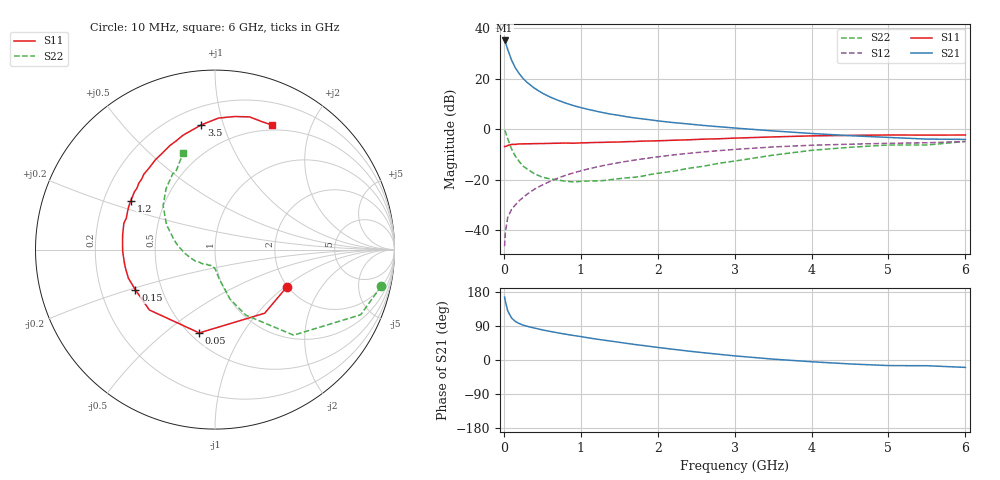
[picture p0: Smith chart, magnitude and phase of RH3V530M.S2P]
! SIEMENS Small Signal Semiconductors
! BFR106
! Si NPN RF Bipolar Junction Transistor in SOT23
! VCE = 3.5 V  IC = 30 mA
! Common Emitter S-Parameters:  August  1996
# GHz  S  MA  R  50
!  f  S11  S21  S12  S22
! GHz  MAG  ANG  MAG  ANG  MAG  ANG  MAG  ANG
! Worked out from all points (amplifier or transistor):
!   36 points, 10 MHz to 6 GHz, reference 50 ohm
!   highest |S21| = 35.1 dB at 10 MHz (marker M1)
!   |S21| within 3 dB of that: start of sweep to 44.24 MHz
!   unconditionally stable (mu >= 1): 306.7 MHz to 2.267 GHz; 5.499141 GHz to 5.503862 GHz
!   at 250 MHz: K = 0.96, MSG = 23.6 dB, |S12| = -27.1 dB
!   at 1.4 GHz: K = 1.06, MAG = 8.3 dB, |S12| = -13.8 dB
!   at 6 GHz: K = 1.00, MSG = 0.4 dB, |S12| = -4.9 dB
!   S11 on the Smith chart (normalised r, x): 10 MHz: 1.97, -1.03; 50 MHz: 0.56, -0.66; 150 MHz: 0.35, -0.21; 1.2 GHz: 0.32, +0.24; 3.5 GHz: 0.31, +0.85; 6 GHz: 0.44, +1.46
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0.01  0.451 -27.6  56.8 165.9  0.0048 83.1  0.9484 -12.4
0.02  0.4497 -52.0  52.58 154.4  0.0091 73.2  0.8891 -24.1
0.05  0.4725 -100.7  37.73 129.8  0.0176 60.0  0.6475 -47.4
0.1  0.4969 -137.4  23.27 111.0  0.0256 56.5  0.4039 -64.8
0.15  0.4969 -153.1  16.27 101.6  0.0316 58.1  0.29 -73.0
0.2  0.5081 -161.7  12.51 96.2  0.0382 61.9  0.2276 -76.0
0.25  0.5094 -168.0  10.05 92.0  0.044 63.6  0.1854 -79.7
0.3  0.5103 -171.8  8.441 89.1  0.051 65.8  0.1629 -82.1
0.4  0.5146 -179.1  6.409 84.1  0.0646 67.6  0.13 -85.6
0.5  0.5164 175.9  5.143 79.6  0.078 68.4  0.1115 -88.2
0.6  0.5208 171.2  4.317 75.6  0.092 68.6  0.1032 -91.3
0.7  0.5242 167.0  3.73 71.7  0.1066 68.3  0.0983 -95.6
0.9  0.5242 160.5  2.931 64.9  0.1348 66.7  0.09 -102.7
1.1  0.5376 153.4  2.444 58.4  0.1628 64.8  0.0937 -112.3
1.2  0.543 149.8  2.261 55.3  0.1763 63.5  0.0939 -117.4
1.6  0.5631 138.9  1.749 43.8  0.2304 58.2  0.1082 -135.8
2.2  0.6002 123.7  1.345 28.3  0.3071 49.5  0.1461 -162.6
2.8  0.6429 109.7  1.111 15.0  0.3745 40.2  0.2105 173.1
3.5  0.699 96.3  0.919 2.3  0.4424 29.6  0.3043 152.7
4.5  0.7493 81.7  0.739 -10.4  0.502 14.7  0.4358 128.7
5.5  0.7593 69.5  0.633 -15.1  0.5354 4.9  0.4841 116.9
6  0.7626 65.6  0.624 -19.5  0.5666 -2.3  0.5688 108.1
